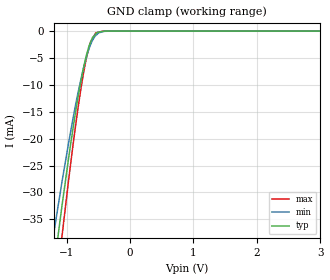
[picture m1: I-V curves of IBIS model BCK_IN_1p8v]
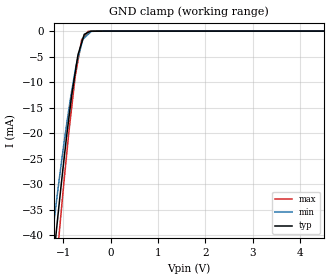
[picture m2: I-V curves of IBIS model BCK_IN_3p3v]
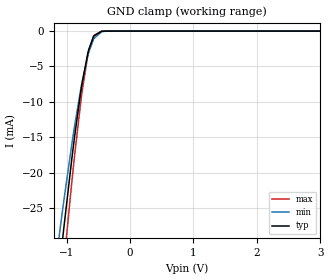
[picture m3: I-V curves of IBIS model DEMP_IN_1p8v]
|Texas Instruments Incorporated
|2VRMS DIRECTPATH Audio Stereo DAC
| Marketing part#   Voltage Range(Digital)   Package-type   #pins
|PCM5101XXX   1.65V to 3.6V   TBD   20
[IBIS Ver]   4.0
[File name]   pcm5101.ibs
[File Rev]   1.0
[Date]   03/15/2011
[Source]   Texas Instruments Incorporated.
   Analog-eLab, HPA
   12500 TI Blvd
   Dallas, TX -75243
   For Support e-mail: elab_ibis@list.ti.com
[Notes]   Revision History:
   1.0: 03/15/2011
   - Initial version of the model
   - Initial Model generated from simulations.
   - Model names with a trailing _1p8v contains the model for
   1.8V (1.65V and 1.95V). Model names with trailing _3p3v
   contains the model for 3.3V (3.0V and 3.6V) operation.
   - Model not matched to measurements
[Disclaimer]
 This product is designed as an aid for customers of Texas Instruments.
 No warranties, either expressed or implied, with respect to this third
 party software (if any) or with respect to its fitness for any
 particular purpose is claimed by Texas Instruments or the author. The
 software (if any) is provided solely on an "as is" basis. The entire
 risk as to its quality and performance is with the customer
[Copyright] (C) Copyright 2011 Texas Instruments Incorporated.
   All rights reserved.
|   PCM5101
[Component]   pcm5101
[Manufacturer] TI
[Package]   | 20 pin  package
| variable   typ   min   max
R_pkg   0.1   NA   NA
L_pkg   1.5nH   NA   NA
C_pkg   0.5pF   NA   NA
|-------------------------PIN------------------------------------------------
[Pin] signal_name  model_name  R_pin  L_pin C_pin
1   CPVDD   POWER   NA   NA   NA
2   CAPP   TERM   NA   NA   NA
3   CPGND   GND   NA   NA   NA
4   CAPM   TERM   NA   NA   NA
5   VNEG   TERM   NA   NA   NA
6   OUTL   TERM   NA   NA   NA
7   OUTR   TERM   NA   NA   NA
8   AVDD   POWER   NA   NA   NA
9   AGND   GND   NA   NA   NA
10   DEMP   DEMP_IN   NA   NA   NA
11   FLT   FLT_IN   NA   NA   NA
12   SCK   SCK_IN   NA   NA   NA
13   BCK   BCK_IN   NA   NA   NA
14   DIN   SCK_IN   NA   NA   NA
15   LRCK   BCK_IN   NA   NA   NA
16   FMT   FLT_IN   NA   NA   NA
17   SXMT   DEMP_IN   NA   NA   NA
18   LDOO   TERM   NA   NA   NA
19   DGND   GND   NA   NA   NA
20   DVDD   POWER   NA   NA   NA
[Pin Mapping]pulldown_ref pullup_ref gnd_clamp_ref power_clamp_ref |ext_ref
1   NC   PWRBUS1   |charge pump power supply
2   GNDBUS1   PWRBUS1   GNDBUS1   PWRBUS1
3   GNDBUS1   NC   |charge pump ground
4   GNDBUS1   PWRBUS1   GNDBUS1   PWRBUS1
5   GNDBUS1   PWRBUS1   GNDBUS1   PWRBUS1
6   GNDBUS2   PWRBUS2   GNDBUS2   PWRBUS2
7   GNDBUS2   PWRBUS2   GNDBUS2   PWRBUS2
8   NC   PWRBUS2   | analog power supply
9   GNDBUS2   NC   | analog ground
10   NC   NC   GNDBUS3   PWRBUS3
11   NC   NC   GNDBUS3   PWRBUS3
12   NC   NC   GNDBUS3   PWRBUS3
13   NC   NC   GNDBUS3   PWRBUS3
14   NC   NC   GNDBUS3   PWRBUS3
15   NC   NC   GNDBUS3   PWRBUS3
16   NC   NC   GNDBUS3   PWRBUS3
17   NC   NC   GNDBUS3   PWRBUS3
18   GNDBUS3   PWRBUS3   GNDBUS3   PWRBUS3
19   GNDBUS3   NC   |digital power supply
20   NC   PWRBUS3   |digital ground
[Model Selector] DEMP_IN
DEMP_IN_3p3v   3.3V DEMP/SXMT input
DEMP_IN_1p8v   1.8V DEMP/SXMT input
[Model Selector] FLT_IN
FLT_IN_3p3v   3.3V FLT/FMT input
FLT_IN_1p8v   1.8V FLT/FMT input
[Model Selector] SCK_IN
SCK_IN_3p3v   3.3V SCK/DIN input
SCK_IN_1p8v   1.8V SCK/DIN input
[Model Selector] BCK_IN
BCK_IN_3p3v   3.3V BCK/LRCK input
BCK_IN_1p8v   1.8V BCK/LRCK input
|   TERM Model
[Model] TERM
Model_type Terminator
C_comp   0   0   0
| variable   typ   min   max
[Voltage Range]   3.3V   3.0V   3.6V
[POWER Clamp Reference]  3.3V   3.0V   3.6V
[GND Clamp Reference]   0.0V   0.0V   0.0V
|Operating Temperature
[Temperature Range]   27   105   -25
| Models and submodels in the file (9): BCK_IN_1p8v (Input), BCK_IN_3p3v (Input), DEMP_IN_1p8v (Input), DEMP_IN_3p3v (Input), FLT_IN_1p8v (Input), FLT_IN_3p3v (Input), SCK_IN_1p8v (Input), SCK_IN_3p3v (Input), TERM (Terminator)
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|   BCK_IN_1p8v
[Model]   BCK_IN_1p8v
Model_type   Input
Vinl = 0.54
Vinh = 1.26
|   typ   min   max
C_comp   1.514291423pF   1.436730626pF   1.542051917pF
[Voltage Range]   1.8   1.65   1.95
[Temperature Range]   27   105   -25
[Power Clamp Reference]   1.8   1.65   1.95
[GND Clamp Reference]   -0   -0   -0
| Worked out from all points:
|   GND clamp passes 1 mA (typ) near -0.57 V on its own axis
[GND Clamp]
|   Voltage   I(typ)   I(min)   I(max)
-1.8V     -103.9mA   -86.97mA   -120.1mA
-1.29V    -52.65mA   -44.58mA   -61.57mA
-1.182V   -42.49mA   -36.24mA   -49.8mA
-1.074V   -32.76mA   -28.25mA   -38.44mA
-974.7mV  -24.27mA   -21.3mA    -28.44mA
-880.4mV  -16.79mA   -15.16mA   -19.63mA
-734.2mV  -6.985mA   -6.98mA    -7.926mA
-686.2mV  -4.486mA   -4.819mA   -4.945mA
-622.6mV  -2.125mA   -2.565mA   -2.05mA
-539.6mV  -557.4uA   -827.2uA   -348.4uA
-296.6mV  -421.6nA   -3.207uA   -166.4nA
3.6V      0A         0A         0A
[POWER Clamp]
|   Voltage   I(typ)   I(min)   I(max)
-1.8V     0A         0A         0A
0V        0A         0A         0A
3.6V      0A         0A         0A
|   BCK_IN_3p3v
[Model]   BCK_IN_3p3v
Model_type   Input
Vinl = 0.99
Vinh = 2.31
|   typ   min   max
C_comp   1.426525397pF   1.374530485pF   1.444284221pF
[Voltage Range]   3.3   3   3.6
[Temperature Range]   27   105   -25
[Power Clamp Reference]   3.3   3   3.6
[GND Clamp Reference]   -0   -0   -0
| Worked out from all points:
|   GND clamp passes 1 mA (typ) near -0.57 V on its own axis
[GND Clamp]
|   Voltage   I(typ)   I(min)   I(max)
-3.3V     -526.5mA   -489.6mA   -552.8mA
-1.223V   -46.27mA   -39.34mA   -54.17mA
-1.139V   -38.52mA   -32.98mA   -45.18mA
-1.078V   -33.07mA   -28.51mA   -38.81mA
-882.5mV  -17.07mA   -15.34mA   -19.81mA
-746.7mV  -8.048mA   -7.686mA   -8.786mA
-689.8mV  -4.65mA    -5.27mA    -5.807mA
-610.8mV  -2.252mA   -2.464mA   -1.67mA
-557.7mV  -638.8uA   -1.348mA   -1.038mA
-475mV    -252.8uA   -630.3uA   -54.69uA
-230.4mV  -11.43uA   -497.9nA   -215.4nA
6.6V      0A         0A         0A
[POWER Clamp]
|   Voltage   I(typ)   I(min)   I(max)
-3.3V     0A         0A         0A
0V        0A         0A         0A
6.6V      0A         0A         0A
|   DEMP_IN_1p8v
[Model]   DEMP_IN_1p8v
Model_type   Input
Vinl = 0.54
Vinh = 1.26
|   typ   min   max
C_comp   1.023635717pF   1.008986379pF   1.039026956pF
[Voltage Range]   1.8   1.65   1.95
[Temperature Range]   27   105   -25
[Power Clamp Reference]   1.8   1.65   1.95
[GND Clamp Reference]   -0   -0   -0
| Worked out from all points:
|   GND clamp passes 1 mA (typ) near -0.58 V on its own axis
[GND Clamp]
|   Voltage   I(typ)   I(min)   I(max)
-1.8V     -97.74mA   -81.51mA   -113.4mA
-1.238V   -44.53mA   -37.64mA   -52.44mA
-1.093V   -31.94mA   -27.34mA   -37.74mA
-1.044V   -27.93mA   -24.07mA   -33.03mA
-919.8mV  -18.28mA   -16.17mA   -21.6mA
-865.8mV  -14.42mA   -13.01mA   -17mA
-768.6mV  -8.212mA   -7.858mA   -9.529mA
-660.6mV  -2.999mA   -3.364mA   -3.244mA
-568.8mV  -690.4uA   -1.063mA   -614.2uA
-450mV    -38.26uA   -112.2uA   -20.73uA
-347.4mV  -1.66uA    -10.08uA   -447nA
3.6V      0A         0A         0A
[POWER Clamp]
|   Voltage   I(typ)   I(min)   I(max)
-1.8V     0A         0A         0A
0V        0A         0A         0A
3.6V      0A         0A         0A
